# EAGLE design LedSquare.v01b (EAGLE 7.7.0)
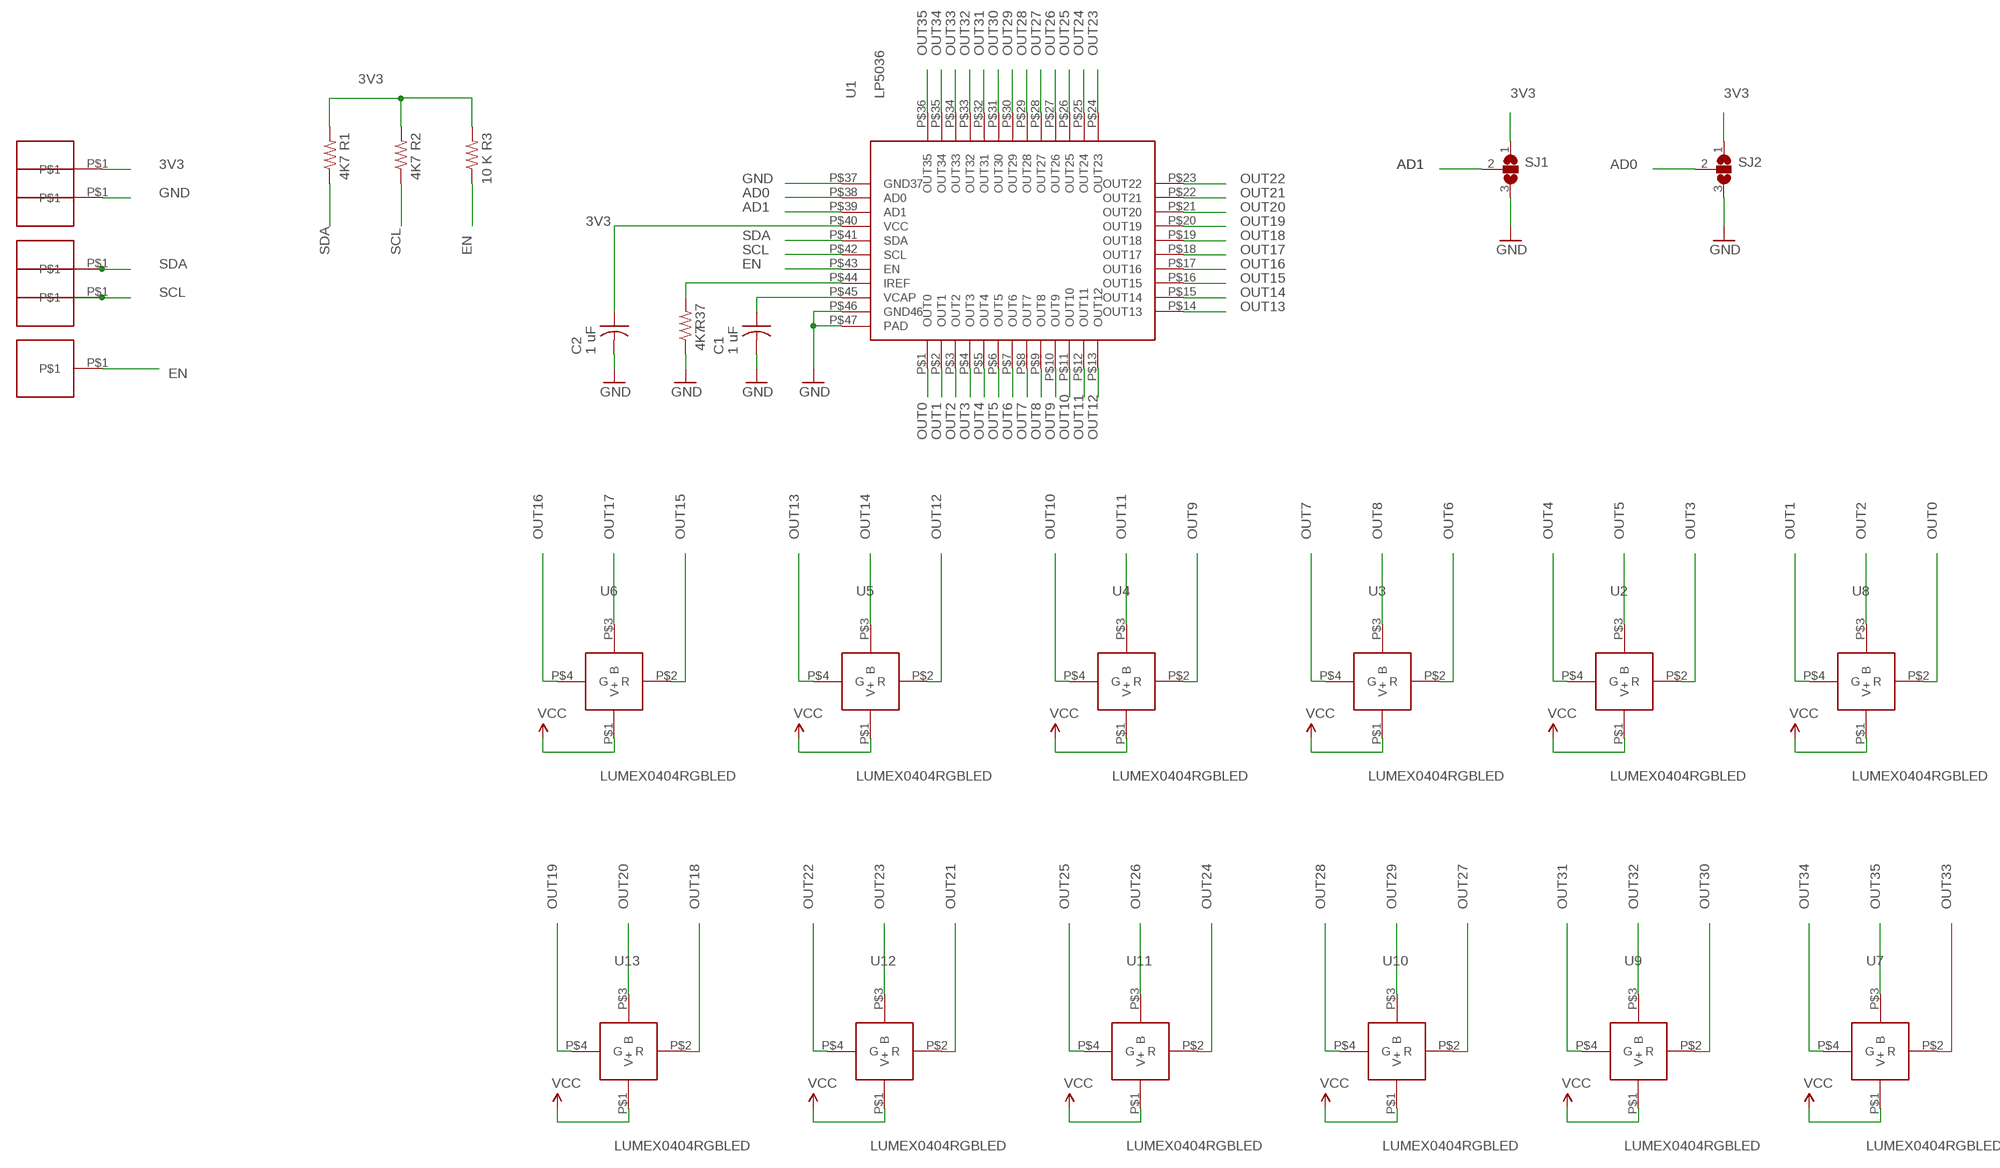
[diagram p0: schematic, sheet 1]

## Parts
C1  1 uF  C-US  [C0402_B]
C2  1 uF  C-US  [C0402_B]
R1  4K7  R-US_  [R0402_B]
R2  4K7  R-US_  [R0402_B]
R3  10 K  R-US_  [R0402_B]
R37  4K7  R-US_  [R0402_B]
SJ1  SJ2W  [SJ_2]
SJ2  SJ2W  [SJ_2]
U1  LP5036  [LP5036]
U2  LUMEX0404RGBLED  [LX0404]
U3  LUMEX0404RGBLED  [LX0404]
U4  LUMEX0404RGBLED  [LX0404]
U5  LUMEX0404RGBLED  [LX0404]
U6  LUMEX0404RGBLED  [LX0404]
U7  LUMEX0404RGBLED  [LX0404]
U8  LUMEX0404RGBLED  [LX0404]
U9  LUMEX0404RGBLED  [LX0404]
U10  LUMEX0404RGBLED  [LX0404]
U11  LUMEX0404RGBLED  [LX0404]
U12  LUMEX0404RGBLED  [LX0404]
U13  LUMEX0404RGBLED  [LX0404]
U$1  HN01  [HN01]
U$2  HN01  [HN01]
U$3  HN01  [HN01]
U$4  HN01  [HN01]
U$9  HN01  [HN01]

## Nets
3V3: C2.1 R1.2 R2.2 R3.2 SJ1.1 SJ2.1 U1.P$40(VCC) U2.P$1(V+) U3.P$1(V+) U4.P$1(V+) U5.P$1(V+) U6.P$1(V+) U7.P$1(V+) U8.P$1(V+) U9.P$1(V+) U10.P$1(V+) U11.P$1(V+) U12.P$1(V+) U13.P$1(V+) U$4.P$1 ; supply symbol labelled VCC
AD0: SJ2.2 U1.P$38(AD0)
AD1: SJ1.2 U1.P$39(AD1)
EN: R3.1 U1.P$43(EN) U$9.P$1
GND: C1.2 C2.2 R37.1 SJ1.3 SJ2.3 U1.P$37(GND37) U1.P$46(GND46) U1.P$47(PAD) U$3.P$1
N$80: R37.2 U1.P$44(IREF)
N$81: C1.1 U1.P$45(VCAP)
OUT0: U1.P$1(OUT0) U8.P$2(R)
OUT1: U1.P$2(OUT1) U8.P$4(G)
OUT2: U1.P$3(OUT2) U8.P$3(B)
OUT3: U1.P$4(OUT3) U2.P$2(R)
OUT4: U1.P$5(OUT4) U2.P$4(G)
OUT5: U1.P$6(OUT5) U2.P$3(B)
OUT6: U1.P$7(OUT6) U3.P$2(R)
OUT7: U1.P$8(OUT7) U3.P$4(G)
OUT8: U1.P$9(OUT8) U3.P$3(B)
OUT9: U1.P$10(OUT9) U4.P$2(R)
OUT10: U1.P$11(OUT10) U4.P$4(G)
OUT11: U1.P$12(OUT11) U4.P$3(B)
OUT12: U1.P$13(OUT12) U5.P$2(R)
OUT13: U1.P$14(OUT13) U5.P$4(G)
OUT14: U1.P$15(OUT14) U5.P$3(B)
OUT15: U1.P$16(OUT15) U6.P$2(R)
OUT16: U1.P$17(OUT16) U6.P$4(G)
OUT17: U1.P$18(OUT17) U6.P$3(B)
OUT18: U1.P$19(OUT18) U13.P$2(R)
OUT19: U1.P$20(OUT19) U13.P$4(G)
OUT20: U1.P$21(OUT20) U13.P$3(B)
OUT21: U1.P$22(OUT21) U12.P$2(R)
OUT22: U1.P$23(OUT22) U12.P$4(G)
OUT23: U1.P$24(OUT23) U12.P$3(B)
OUT24: U1.P$25(OUT24) U11.P$2(R)
OUT25: U1.P$26(OUT25) U11.P$4(G)
OUT26: U1.P$27(OUT26) U11.P$3(B)
OUT27: U1.P$28(OUT27) U10.P$2(R)
OUT28: U1.P$29(OUT28) U10.P$4(G)
OUT29: U1.P$30(OUT29) U10.P$3(B)
OUT30: U1.P$31(OUT30) U9.P$2(R)
OUT31: U1.P$32(OUT31) U9.P$4(G)
OUT32: U1.P$33(OUT32) U9.P$3(B)
OUT33: U1.P$34(OUT33) U7.P$2(R)
OUT34: U1.P$35(OUT34) U7.P$4(G)
OUT35: U1.P$36(OUT35) U7.P$3(B)
SCL: R2.1 U1.P$42(SCL) U$1.P$1
SDA: R1.1 U1.P$41(SDA) U$2.P$1

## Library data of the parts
C1 C2 = Spark:C-US: Capacitor
R1-R3 R37 = Spark:R-US_: 0402 Resistor
SJ1 SJ2 = jumper:SJ2W: SMD solder JUMPER
U1 = Kris:LP5036: LP5036RJVR 12 x 3 rgb led driver http://www.ti.com/lit/ds/symlink/lp5036.pdf
U2-U13 = Kris:LUMEX0404RGBLED: Lumex 0404 rgb leds
U$1-U$4 U$9 = PWSONN6:HN01

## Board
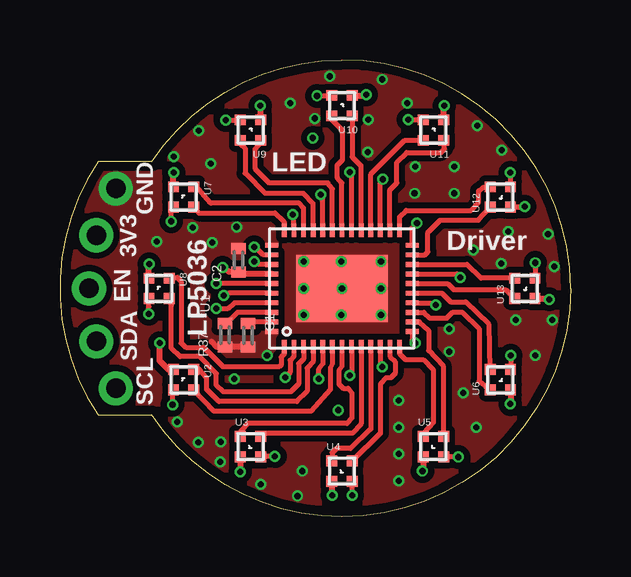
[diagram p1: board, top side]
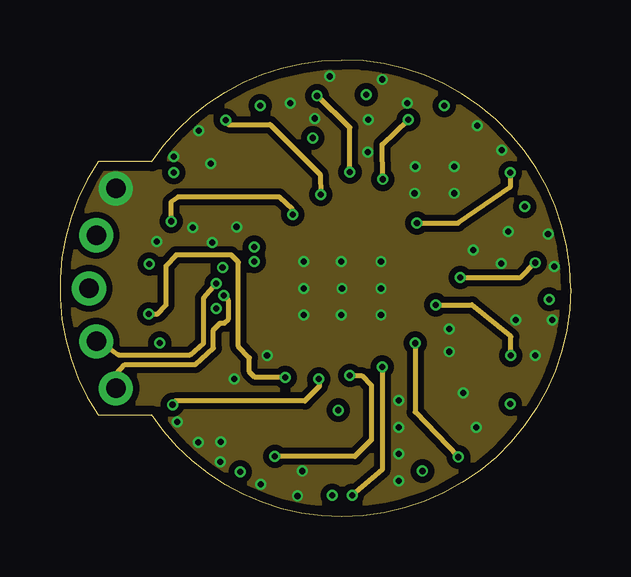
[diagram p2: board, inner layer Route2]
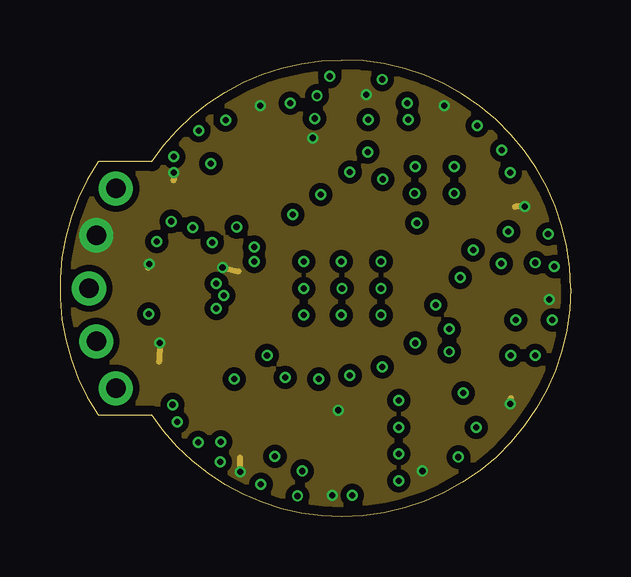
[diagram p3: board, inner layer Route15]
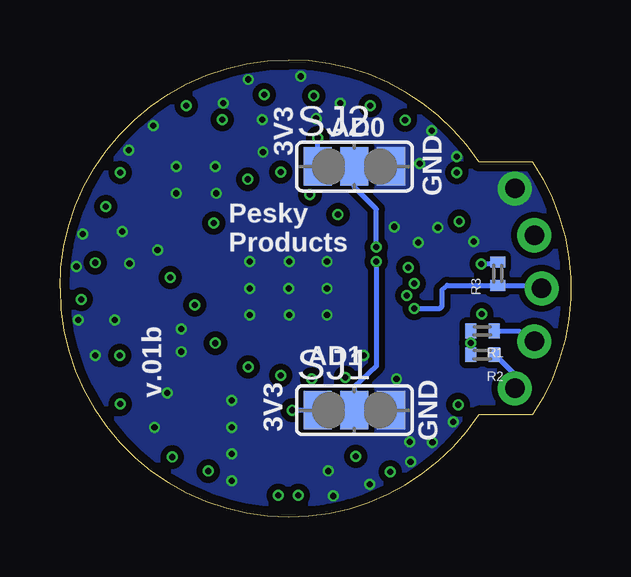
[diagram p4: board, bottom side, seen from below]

Size 21.27 x 19.05 mm. Coordinates in mm from the lower left corner, seen from the top.
Outline: 3.82,14.81 1.59,14.81 arc67 1.59,4.24 3.82,4.24 arc56 11.75,0 arc90 21.27,9.52 arc90 11.75,19.05 arc56 3.82,14.81
Copper layers (1*2*15*16): Top 0.035559375mm / dielectric 0.17018125mm / Route2 0.01778125mm / dielectric 47mil / Route15 0.01778125mm / dielectric 0.17018125mm / Bottom 0.035559375mm
Design rules "OSHPark-4layer *": minimum track width 5mil, minimum drill 10mil, track to track 5mil, track to pad 5mil, pad to pad 5mil, via to via 5mil, smd to smd 5mil, copper to edge 15mil, drill to drill 6mil, minimum pad ring 4mil, minimum via ring 4mil, stop-mask expansion 4mil, vias tented up to drill 20mil, thermal gap 10mil

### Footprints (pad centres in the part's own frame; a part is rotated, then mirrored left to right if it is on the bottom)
C0402_B = smd 0.457 x 0.61: 1 -0.483,0; 2 0.483,0
R0402_B = smd 0.457 x 0.61: 1 -0.483,0; 2 0.483,0
SJ_2 = smd 1.168 x 1.6: 1 -1.524,0; 2 0,0; 3 1.524,0
LP5036 = smd 0.55 x 0.2: P$1 -2.425,2.4; P$2 -2.425,2; P$3 -2.425,1.6; P$4 -2.425,1.2; P$5 -2.425,0.8; P$6 -2.425,0.4; P$7 -2.425,0; P$8 -2.425,-0.4; P$9 -2.425,-0.8; P$10 -2.425,-1.2; P$11 -2.425,-1.6; P$12 -2.425,-2; P$13 -2.425,-2.4; P$24 2.425,-2.4; P$25 2.425,-2; P$26 2.425,-1.6; P$27 2.425,-1.2; P$28 2.425,-0.8; P$29 2.425,-0.4; P$30 2.425,0; P$31 2.425,0.4; P$32 2.425,0.8; P$33 2.425,1.2; P$34 2.425,1.6; P$35 2.425,2; P$36 2.425,2.4 | smd 0.2 x 0.55: P$14 -1.8,-2.925; P$15 -1.4,-2.925; P$16 -1,-2.925; P$17 -0.6,-2.925; P$18 -0.2,-2.925; P$19 0.2,-2.925; P$20 0.6,-2.925; P$21 1,-2.925; P$22 1.4,-2.925; P$23 1.8,-2.925; P$37 1.8,2.925; P$38 1.4,2.925; P$39 1,2.925; P$40 0.6,2.925; P$41 0.2,2.925; P$42 -0.2,2.925; P$43 -0.6,2.925; P$44 -1,2.925; P$45 -1.4,2.925; P$46 -1.8,2.925 | smd 2.8 x 3.8: P$47 0,0
LX0404 = smd 0.45 x 0.45: P$1 -0.425,-0.425; P$2 -0.425,0.425; P$3 0.425,0.425; P$4 0.425,-0.425
HN01 = drill 0.813 pad 1.422: P$1 0,0

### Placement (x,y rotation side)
C1  7.84,7.57 270 top
C2  7.43,10.69 90 top
R1  3.67,7.75 180 bottom
R2  3.67,6.76 180 bottom
R3  3.04,10.13 90 bottom
R37  6.87,7.57 90 top
SJ1  9.01,4.45 0 bottom
SJ2  9.01,14.61 0 bottom
U1  11.75,9.52 90 top
U2  5.15,5.72 270 top
U3  7.94,2.93 0 top
U4  11.75,1.91 0 top
U5  15.56,2.93 0 top
U6  18.35,5.72 90 top
U7  5.15,13.34 270 top
U8  4.13,9.52 270 top
U9  7.94,16.12 180 top
U10  11.75,17.14 180 top
U11  15.56,16.12 180 top
U12  18.35,13.34 90 top
U13  19.37,9.52 90 top
U$1  2.33,5.36 0 top
U$2  1.51,7.32 0 top
U$3  2.33,13.69 0 top
U$4  1.51,11.73 0 top
U$9  1.21,9.52 0 top

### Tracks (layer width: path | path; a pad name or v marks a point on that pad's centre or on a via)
3V3  (via drill 0.25)
  Top 0.254: U1.P$40 7.55,10.12 C2.1 7.05,10.21 v6.77,10.39 | U9.P$1 8.36,17.13 v8.35,17.14 | U10.P$1 12.85,17.57 v12.77,17.6 | U11.P$1 15.98,17.08 v16.02,17.14 | U12.P$1 18.79,12.91 v19.37,12.93 | U13.P$1 20.35,9.1 v20.39,9.07 | U6.P$1 18.77,4.89 v18.76,4.7 | U5.P$1 15.13,1.97 v15.1,1.91 | U4.P$1 11.32,0.96 v11.34,0.89 | U8.P$1 3.7,10.52 v3.72,10.54 | U7.P$1 4.73,14.24 v4.74,14.35 | U3.P$1 7.51,1.84 v7.51,1.88 | U2.P$1 4.52,6.14 4.15,6.5 v4.15,7.25
  Route15 0.203: v11.6,4.45 11.7,4.5
  Route15 0.254: v6.77,10.39 7.43,10.24 | v8.35,17.14 8.35,17.2 8.4,17.14 | v12.77,17.6 12.71,17.55 12.66,17.6 | v16.02,17.14 15.97,17.04 | v19.37,12.93 18.96,12.93 | v20.39,9.07 20.28,9.07 20.33,9.12 | v18.76,4.7 18.79,4.95 | v15.1,1.91 15.15,1.96 15.1,2.01 | v11.34,0.89 11.29,0.89 | v4.15,7.25 4.13,6.48 | v3.72,10.54 3.77,10.49 3.67,10.39 | v4.74,14.35 4.74,14.02 | v7.51,1.88 7.51,2.46
  Bottom 0.203: SJ2.1 v10.53,15.8 | SJ1.1 v11.6,4.45 11.7,4.45 | R3.2 3.34,10.54 v3.72,10.54 | R2.2 4.18,7.23 v4.15,7.25
  Bottom 0.254: R1.2 R2.2
  pour Route15 (isolate 0.254, no thermals): -0.95,22.22 24.45,22.22 24.45,-3.17 -0.95,-3.17
AD0  (via drill 0.25)
  Top 0.203: U1.P$38 8.47,10.93 8.14,11.25 v8.09,11.25
  Bottom 0.203: v8.09,11.25 8.09,12.83 9.01,13.74 SJ2.2
AD1  (via drill 0.25)
  Top 0.203: U1.P$39 8.26,10.52 v8.09,10.64
  Bottom 0.127: SJ1.2 7.53,4.45
  Bottom 0.203: v8.09,10.64 8.09,6.27 9.01,5.41 SJ1.2
EN  (via drill 0.25)
  Top 0.203: U1.P$43 7.26,8.93 7,8.69 v6.52,8.69
  Bottom 0.203: v6.52,8.69 5.45,8.69 5.35,8.79 5.35,9.47 5.15,9.65 R3.1 1.34,9.65 U$9.P$1
GND  (via drill 0.25)
  Top 0.254: C1.2 6.52,7.09 6.31,7.29
  other vias: 11.75,9.52 8.63,6.73 10.15,10.64 11.72,10.64 13.38,10.64 13.38,8.41 13.38,9.52 11.72,8.41 10.15,8.41 10.15,9.52 5.76,3.1 9.9,0.86 14.11,1.5 14.11,3.73 17.34,3.73 14.11,2.62 14.11,4.85 19.8,6.73 20.51,8.2 18.99,8.2 20.59,10.44 18.68,11.89 16.22,7.82 16.22,6.88 17.21,11.13 17.39,16.31 18.4,15.29 7.36,12.09 4.74,15.01 6.29,14.73 11.24,18.36 9.59,17.25 13.43,18.24 14.47,17.25 14.8,14.61 16.42,13.49 16.42,14.61 14.77,13.49 12.84,16.56 12.82,15.21 6.34,11.43 5.53,12.07 4.03,11.48 10.61,16.61 10.1,1.91 20.34,11.79 18.38,10.57 6.67,2.29 4.89,3.96 5.78,16.1 7.25,5.74 16.8,5.16 6.7,3.12 8.37,1.35
  pour Bottom (isolate 0.254, no thermals): -0.95,22.22 24.45,22.22 24.45,-3.17 -0.95,-3.17
  pour Top (isolate 0.254, no thermals): -0.95,22.22 24.45,22.22 24.45,-3.17 -0.95,-3.17
  pour Route2 (isolate 0.254, no thermals): -0.95,22.22 24.45,22.22 24.45,-3.17 -0.95,-3.17
N$2
  Bottom 0.127: 9.01,14.61 7.53,14.61
N$80
  Top 0.203: U1.P$44 7.4,8.52 6.87,8 6.75,8 R37.2
N$81
  Top 0.203: U1.P$45 7.99,8.12 C1.1
OUT0
  Top 0.203: U1.P$1 9.35,6.8 9.21,6.66 9.21,6.33 9.13,6.25 6.8,6.25 5.98,7.06 5.25,7.06 5.04,7.24 5.04,9.8 4.89,9.98 4.59,9.98 U8.P$2
OUT1  (via drill 0.25)
  Top 0.203: U1.P$2 9.75,6.69 9.59,6.53 9.59,6.02 v9.39,5.82 | v3.7,8.46 3.7,8.76 U8.P$4
  Route2 0.203: v9.39,5.82 8.12,5.82 7.89,6.05 7.89,6.63 7.43,7.11 7.43,10.62 7.13,10.92 4.84,10.92 4.41,10.46 4.41,8.81 4.08,8.46 v3.7,8.46
OUT2
  Top 0.203: U1.P$3 10.15,6.58 9.95,6.38 9.95,5.54 9.62,5.21 6.8,5.21 6.52,5.49 6.52,5.97 5.83,6.68 4.99,6.68 4.64,7.01 4.64,8.83 U8.P$3
OUT3
  Top 0.203: U1.P$4 10.55,6.47 10.3,6.2 10.3,5.23 9.87,4.8 6.62,4.8 6.11,5.31 6.11,5.79 5.81,6.15 5.66,6.15 U2.P$2
OUT4  (via drill 0.25)
  Top 0.203: U1.P$5 10.95,6.39 10.78,6.17 v10.78,5.74 | v4.69,4.67 4.69,5.15 U2.P$4
  Route2 0.203: v10.78,5.74 10.81,5.44 10.2,4.83 4.79,4.83 v4.69,4.67
OUT5
  Top 0.203: U1.P$6 11.35,6.38 11.27,6.22 11.27,5.31 10.45,4.39 6.42,4.39 U2.P$3
OUT6
  Top 0.203: U1.P$7 11.75,6.27 11.62,6.1 11.62,5.54 11.8,5.36 12,5.36 12.16,5.16 12.16,4.12 11.95,3.89 7.81,3.89 7.53,3.58 7.56,3.4 U3.P$2 7.53,3.37
OUT7  (via drill 0.25)
  Top 0.203: U1.P$8 12.15,6.01 v12.08,5.89 | v8.96,2.52 U3.P$4
  Route2 0.203: 9.03,2.57 v8.96,2.52 12.28,2.52 12.97,3.2 12.97,5.49 12.56,5.89 v12.08,5.89
OUT8
  Top 0.203: U3.P$3 8.54,3.48 12.18,3.48 12.55,3.87 U1.P$9
OUT9
  Top 0.203: U4.P$2 11.34,2.35 11.34,2.67 11.52,2.84 12.11,2.84 12.95,3.66 U1.P$10
OUT10  (via drill 0.25)
  Top 0.203: U1.P$11 13.35,6.3 v13.43,6.25 | v12.18,0.89 12.18,1.47 U4.P$4
  Route2 0.203: v13.43,6.25 13.43,1.96 v12.18,0.89
OUT11
  Top 0.203: 12.19,2.31 U4.P$3 13.35,3.48 13.35,5.54 13.58,5.79 13.78,5.79 13.96,5.97 13.96,6.48 13.75,6.69 U1.P$12
OUT12
  Top 0.203: U1.P$13 14.15,6.8 14.39,6.55 15.13,6.55 15.56,6.12 15.56,3.94 15.13,3.48 15.13,3.36 U5.P$2
OUT13  (via drill 0.25)
  Top 0.203: U1.P$14 14.67,7.36 v14.8,7.24 | v16.6,2.49 16,2.49 U5.P$4
  Route2 0.203: v14.8,7.24 14.8,4.37 v16.6,2.49
OUT14
  Top 0.203: U1.P$15 14.98,8.12 15.36,7.77 15.36,6.93 15.97,6.3 15.97,3.37 U5.P$3
OUT15
  Top 0.203: U1.P$16 15.16,8.52 15.41,8.28 16.12,8.28 16.37,8.53 16.75,8.53 17.46,7.85 17.46,5.66 U6.P$2
OUT16  (via drill 0.25)
  Top 0.203: U1.P$17 15.58,8.93 v15.66,8.84 | v18.79,6.73 18.79,6.15 U6.P$4
  Route2 0.203: v15.66,8.84 17.16,8.84 18.79,7.52 v18.79,6.73
OUT17
  Top 0.203: U1.P$18 15.91,9.32 16.27,8.97 16.91,8.97 17.88,8.02 U6.P$3
OUT18
  Top 0.203: U1.P$19 16.15,9.73 16.4,9.47 18.57,9.47 U13.P$2
OUT19  (via drill 0.25)
  Top 0.203: U1.P$20 16.53,10.12 v16.68,9.98 | v19.8,10.59 19.8,9.96 U13.P$4
  Route2 0.203: v16.68,9.98 19.19,9.98 v19.8,10.59
OUT20
  Top 0.203: U1.P$21 16.96,10.52 17.53,9.95 U13.P$3
OUT21
  Top 0.203: U1.P$22 15.21,10.93 15.33,11.05 15.33,11.86 15.84,12.37 17.43,12.37 U12.P$2
OUT22  (via drill 0.25)
  Top 0.203: U1.P$23 14.67,12.04 v14.87,12.24 | v18.76,14.35 18.76,13.87 U12.P$4
  Route2 0.203: v14.87,12.24 16.58,12.24 18.76,13.74 v18.76,14.35
OUT23
  Top 0.203: U1.P$24 14.15,12.51 14.42,12.78 17.13,12.78 17.44,13.11 17.44,13.59 17.64,13.74 17.89,13.74 U12.P$3
OUT24
  Top 0.203: U11.P$2 16.02,15.67 16.02,15.34 15.86,15.19 14.44,15.19 14.04,14.78 14.04,13.92 13.75,13.63 U1.P$25
OUT25  (via drill 0.25)
  Top 0.203: U1.P$26 13.35,13.94 v13.45,14.07 | v14.52,16.56 15.12,16.56 U11.P$4
  Route2 0.203: v13.45,14.07 13.43,15.52 v14.52,16.56
OUT26
  Top 0.203: U1.P$27 12.95,14.28 14.37,15.7 U11.P$3
OUT27
  Top 0.203: U1.P$28 12.55,14.63 12.17,15 U10.P$2
OUT28  (via drill 0.25)
  Top 0.203: U1.P$29 12.15,14.2 v12.08,14.38 | v10.71,17.55 11.31,17.55 U10.P$4
  Route2 0.203: v12.08,14.38 12.08,16.23 v10.71,17.55
OUT29
  Top 0.203: U1.P$30 11.75,13.92 11.55,14.15 11.55,14.66 11.77,14.88 11.77,16.1 11.34,16.54 11.34,16.7 U10.P$3
OUT30
  Top 0.203: U1.P$31 11.35,13.68 11.17,13.92 8.73,13.92 8.12,14.53 8.12,15.34 8.35,15.6 8.35,15.68 U9.P$2
OUT31  (via drill 0.25)
  Top 0.203: U1.P$32 10.95,13.32 v10.86,13.44 | v6.9,16.54 U9.P$4
  Route2 0.203: v6.9,16.54 7,16.36 8.75,16.36 10.84,14.27 v10.86,13.44
OUT32
  Top 0.203: U1.P$33 10.55,13.06 10.15,13.49 8.55,13.49 7.71,14.33 7.71,15.37 7.51,15.57 U9.P$3
OUT33
  Top 0.203: U1.P$34 10.15,12.24 10.15,12.37 10.15,12.88 9.97,13.08 6.29,13.08 6.01,13.39 5.7,13.77 U7.P$2
OUT34  (via drill 0.25)
  Top 0.203: U1.P$35 9.75,12.49 v9.69,12.6 | v4.64,12.32 4.64,12.87 U7.P$4
  Route2 0.203: v9.69,12.6 9.69,12.8 9.13,13.34 4.92,13.34 4.62,13.11 4.62,12.38 v4.64,12.32
OUT35
  Top 0.203: U1.P$36 9.35,12.28 8.96,12.68 5.78,12.68 U7.P$3
SCL  (via drill 0.25)
  Top 0.203: U1.P$42 8.65,9.32 7.03,9.32 v6.82,9.22
  Route2 0.203: v6.82,9.22 7.03,9.02 7.03,8.25 6.85,8.08 6.67,8.08 6.39,7.8 6.39,7.04 5.63,6.35 2.71,6.35 2.34,5.96 2.34,5.38 U$1.P$1
  Bottom 0.203: R2.1 3.14,6.76 2.38,6 2.38,5.41 U$1.P$1
SDA  (via drill 0.25)
  Top 0.203: U1.P$41 v6.52,9.73
  Route2 0.203: v6.51,9.73 v6.52,9.73 5.98,9.11 5.98,7.24 5.42,6.76 2.43,6.76 1.97,7.09 U$2.P$1
  Bottom 0.203: R1.1 2.15,7.75 U$2.P$1

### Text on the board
tPlace: LED | GND | 3V3 | Driver | EN | LP5036 | SDA | SCL
bPlace: AD0 | 3V3 | GND | Pesky / Products | v.01b | AD1 | GND | 3V3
